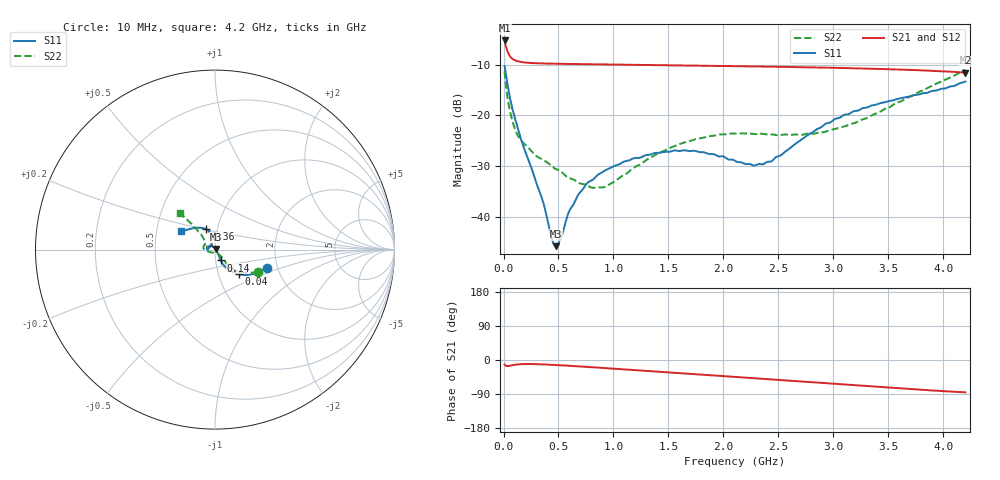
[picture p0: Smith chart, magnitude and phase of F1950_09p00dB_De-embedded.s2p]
! Integrated Device Technology
! Corporate Headquarters
! 6024 Silver Creek Valley Road
! San Jose, CA 95138  USA
! Phone:  1-408-284-8200
! Toll Free:  1-800-223-1366
! Webpage:  http://www.idt.com/
! Timing and RF Division
! 515 Groton Road, Suite 102
! Westford, MA 01886-6024
! Device:  F1950
! Description: 7-bit 0.25 dB Digital Step Attenuator
! Frequency:  150.0 -  4000.00 MHz
! Package:  4x4 mm Thin QFN Plastic Package: 24 pin
! Ports:  2 RF, 12 DC
!  Pin  1  = D0
!  Pin  2  = VDD
!  Pin  3  = Vmode
!  Pin  4  = GND
!  Pin  5  = RF1  =  Port 1
!  Pin  6  = GND
!  Pin  7  = GND
!  Pin  8  = GND
!  Pin  9  = GND
!  Pin 10  = GND
!  Pin 11  = GND
!  Pin 12  = GND
!  Pin 13  = GND
!  Pin 14  = RF2  =  Port 2
!  Pin 15  = GND
!  Pin 16  = LE
!  Pin 17  = CLK
!  Pin 18  = DATE
!  Pin 19  = D6
!  Pin 20  = D5
!  Pin 21  = D4
!  Pin 22  = D3
!  Pin 23  = D2
!  Pin 24  = D1
! State:  36
! Atten State:  9.00 dB
! Voltage:  +5.00 Volts
! Current:  Not Measured mA
! Data:  The device was measured on a the F195X evaluation board which has
!  individual transmission lines to the RF pins.  Data was collected
!  using a calibrated network analyzer.  The evaluation board was
!  de-embedded using a TRL calibration technique.
!  The reference plane is the edge of the package pin.
! Misc:  Board 2019
!  Action Tracker AT0250
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# GHz S dB R 50
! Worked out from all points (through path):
!   420 points, 10 MHz to 4.2 GHz, reference 50 ohm
!   highest |S21| = -5.26 dB at 10 MHz (marker M1); lowest = -11.6 dB at 4.2 GHz (marker M2)
!   group delay of S21, straight-line fit = 53.4 ps
!   lowest |S11| = -45.7 dB at 480 MHz (marker M3), VSWR 1.01, Z = 50.4 + j0.349 ohm
!   |S11| at or under -10 dB: start of sweep to end of sweep
!   |S22| runs from -34.2 to -11.0 dB; largest |S21 - S12| = 0.00041
!   S11 on the Smith chart (normalised r, x): 10 MHz: 1.75, -0.39; 40 MHz: 1.25, -0.36; 140 MHz: 1.06, -0.13; 3.36 GHz: 0.88, +0.20; 4.2 GHz: 0.67, +0.15
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0.01  -10.32 -19.4  -5.26 -12.0  -5.26 -12.0  -11.34 -28.1
0.04  -14.36 -45.7  -7.61 -16.1  -7.61 -16.1  -16.96 -48.1
0.09  -19.48 -60.4  -9.00 -13.2  -9.00 -13.3  -21.79 -49.3
0.14  -23.31 -62.5  -9.41 -11.3  -9.41 -11.3  -24.31 -48.1
0.35  -36.35 -41.7  -9.78 -11.5  -9.78 -11.4  -28.63 -50.5
0.44  -44.30 -3.3  -9.83 -12.7  -9.83 -12.7  -30.02 -52.3
0.48  -45.74 42.2  -9.84 -13.3  -9.84 -13.3  -30.60 -56.0
0.52  -44.15 78.0  -9.86 -13.9  -9.86 -13.9  -30.97 -57.5
0.6  -38.71 108.3  -9.88 -15.3  -9.88 -15.3  -32.37 -64.9
0.71  -34.83 122.7  -9.92 -17.3  -9.92 -17.3  -33.47 -78.2
0.81  -32.69 130.8  -9.94 -19.1  -9.94 -19.1  -34.24 -94.9
0.93  -30.75 139.8  -9.98 -21.4  -9.98 -21.4  -34.01 -117.3
1.41  -27.37 166.9  -10.11 -30.7  -10.11 -30.8  -27.40 -167.3
1.73  -26.97 176.1  -10.20 -37.1  -10.20 -37.1  -24.77 -179.5
2.11  -29.01 167.8  -10.31 -44.8  -10.31 -44.8  -23.61 170.4
2.28  -29.90 148.5  -10.37 -48.2  -10.36 -48.2  -23.68 166.1
2.43  -29.08 128.6  -10.42 -51.1  -10.42 -51.2  -23.74 161.9
2.81  -23.33 104.1  -10.55 -58.9  -10.55 -59.0  -23.64 147.7
3.09  -19.98 106.4  -10.68 -64.7  -10.67 -64.7  -22.24 139.8
3.36  -17.99 114.8  -10.83 -70.1  -10.82 -70.2  -19.85 134.3
3.51  -17.15 120.0  -10.92 -73.1  -10.91 -73.1  -18.38 132.7
4.2  -13.34 151.3  -11.58 -85.3  -11.58 -85.4  -11.00 134.1
